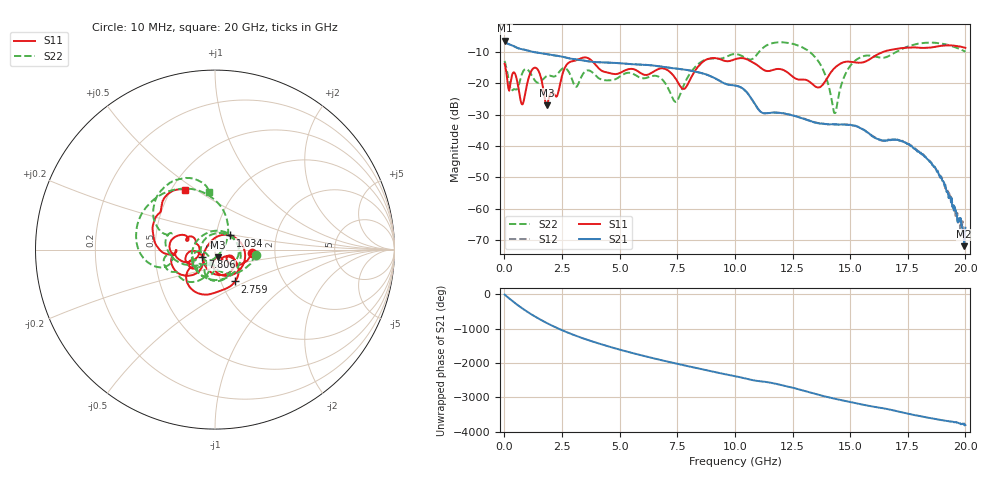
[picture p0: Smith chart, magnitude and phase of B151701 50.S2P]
!  2-Port S-parameters saved by WinCal
! VAR MeasName=S-Parameters (CALIBRATED_DATA) read from VNA (N5244A)
! VAR MeasDate=2015-12-24 19:15:24
! VAR NAME=B151701 50
! VAR FILENAME=B151701 50.S2P
! VAR DATE=2015-12-24 19:15:24
! VAR PHYS_PORTS=1,3
# Hz S DB R 50
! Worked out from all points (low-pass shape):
!   801 points, 10 MHz to 20 GHz, reference 50 ohm
!   highest |S21| = -6.31 dB at 10 MHz (marker M1); lowest = -72.0 dB at 19.95 GHz (marker M2)
!   |S21| within 3 dB of the highest: start of sweep to 918.4 MHz
!   lowest |S11| = -27.0 dB at 1.834 GHz (marker M3), VSWR 1.09, Z = 51.4 - j4.32 ohm
!   |S11| at or under -10 dB: start of sweep to 16.41 GHz
!   |S22| runs from -29.5 to -6.8 dB; largest |S21 - S12| = 0.0031
!   S11 on the Smith chart (normalised r, x): 10 MHz: 1.52, -0.07; 1.034 GHz: 1.17, +0.19; 2.759 GHz: 1.17, -0.43; 7.806 GHz: 0.87, -0.07; 20 GHz: 0.59, +0.45
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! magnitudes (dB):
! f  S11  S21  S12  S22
! 10 MHz  -13.7  -6.3  -6.3  -12.8
! 184.9 MHz  -21.8  -7.4  -7.4  -18.7
! 359.8 MHz  -16.8  -7.9  -7.9  -22.1
! 759.6 MHz  -26.7  -9.1  -9.1  -17.0
! 1.034 GHz  -18.7  -9.5  -9.5  -15.8
! 1.434 GHz  -15.4  -10.2  -10.2  -19.8
! 1.834 GHz  -27.0  -10.6  -10.6  -17.6
! 2.759 GHz  -13.6  -11.9  -11.9  -15.9
! 3.358 GHz  -11.8  -12.6  -12.6  -17.6
! 6.682 GHz  -15.4  -14.5  -14.5  -17.8
! 7.406 GHz  -18.3  -15.2  -15.2  -25.8
! 7.806 GHz  -21.7  -15.6  -15.6  -20.2
! 8.706 GHz  -12.6  -17.0  -17.0  -12.5
! 10.01 GHz  -12.3  -20.7  -20.7  -10.6
! 11.18 GHz  -15.3  -29.4  -29.3  -8.9
! 13.35 GHz  -20.1  -32.2  -32.1  -10.6
! 14.33 GHz  -15.1  -33.2  -33.1  -29.5
! 15.15 GHz  -13.2  -33.5  -33.5  -13.1
! 16.68 GHz  -9.4  -38.0  -38.1  -11.2
! 18.6 GHz  -8.4  -46.3  -45.9  -7.0
! 19.95 GHz  -8.5  -72.0  -67.6  -9.7
! 20 GHz  -8.6  -66.1  -67.5  -9.8
